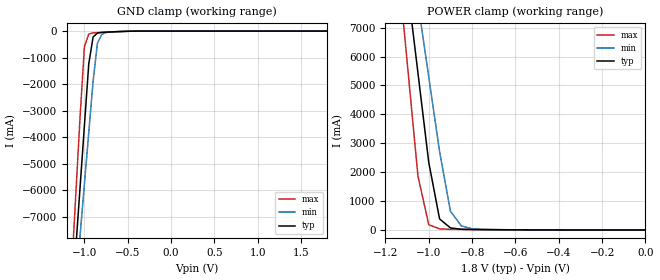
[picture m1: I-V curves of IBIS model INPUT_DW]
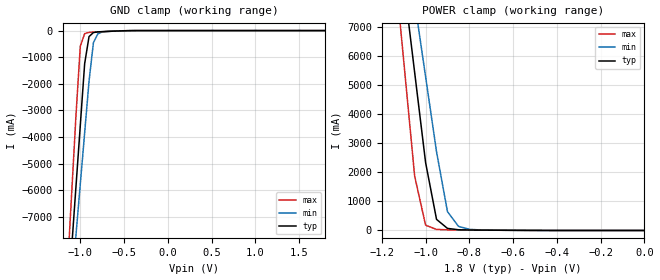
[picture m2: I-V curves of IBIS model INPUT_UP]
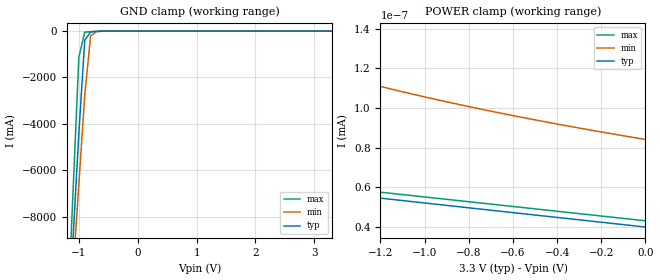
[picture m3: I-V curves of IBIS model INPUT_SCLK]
|   PERICOM SEMICONDUCTOR CORP
|   IBIS Model of PI6CG18801
|   Product Family: 6CG
|   TQFN 48-Pins (ZL) Package
[IBIS Ver] 3.2
[Comment char] |_char
[File Name] pi6cg18801_zl_reva.ibs
[File Rev] 1.0
[Source] File originated at Pericom Semiconductor Corp.
[Date] 12/20/16
[Disclaimer] (C) Copyright PERICOM Semiconductor Corporation
   All rights reserved
  Pericom Semiconductor Corporation hereby grants the user of
  this IBIS model a non-exclusive,nontransferable license to
  use this IBIS model under the following terms.
  This IBIS model is provided on an "AS IS" basis and Pericom
  makes absolutely no warranty with respect to the information
  contained herein. PERICOM DISCLAIMS AND CUSTOMER WAIVES ALL
  WARRANTIES,EXPRESSED OR IMPLIED,INCLUDING WARRANTIES OF
  MERCHANTABILITY OR FITNESS FOR A PARTICULAR PURPOSE. The
  entire risk as to quality and performance is with the customer.
  Accordingly,in no event shall the company be liable for any
  damages,whether in contract or tort,including any lost
  profits or other incidental,consequential,exemplary,or
  punitive damages arising out of the use or application of the
  IBIS model provided in this package. Further,Pericom reserves
  the right to make changes without notice to any product herein
  to improve reliability,function,or design. Pericom does not
  convey any license under patent rights or any other intellectual
  property rights,including those of third parties.
  The user is granted this license only to use the IBIS model
  and is not granted rights to sell,load,rent,lease or license
  the IBIS model in whole or in part,or in modified form to anyone
  other than user. User may modify the IBIS model to suit its specific
  application but rights to derivative works and such modifications
  shall belong to Pericom.
  Pericom is not obligated to provide maintenance or support
  for the licensed IBIS model.
  Contact Pericom at ATTN: APPLICATION ENGINEERING / IBIS MODELS
  1545 Barber Lane Milpitas,CA 95035 USA.
[Component] PI6CG18801
[Manufacturer] Pericom Semiconductor Corp.
[Package]
| Variable   typ   min   max
R_pkg   0.03902ohm   0.02922ohm   0.04882ohm
L_pkg   0.79998nH   0.76828nH   0.83168nH
C_pkg   0.19606pF   0.17176pF   0.22036pF
[Pin]  signal_name   model_name   R_pin   L_pin   C_pin
1   SS_EN_TRI   INPUT_DW   0.04882   0.83168nH   0.22036pF
2   GND_XTAL   GND   0.04490   0.81900nH   0.21064pF
3   XTAL_IN/CLK   NC   0.04098   0.80632nH   0.20092pF
4   XTAL_OUT   NC   0.03706   0.79364nH   0.19120pF
5   VDD_OSC   POWER   0.03314   0.78096nH   0.18148pF
6   VDD_REFOUT   POWER   0.02922   0.76828nH   0.17176pF
7   SDAR/REFOUT   REF_OUT   0.02922   0.76828nH   0.17176pF
8   GND_REFOUT   GND   0.03314   0.78096nH   0.18148pF
9   GND_DIG   GND   0.03706   0.79364nH   0.19120pF
10   SCLK   INPUT_SCLK   0.04098   0.80632nH   0.20092pF
11   SDATA   IO   0.04490   0.81900nH   0.21064pF
12   VDD_DIG   POWER   0.04882   0.83168nH   0.22036pF
13   VDDO   POWER   0.04882   0.83168nH   0.22036pF
14   OE0#   INPUT_DW   0.04490   0.81900nH   0.21064pF
15   Q0+   HCSL_OUT   0.04098   0.80632nH   0.20092pF
16   Q0-   HCSL_OUT   0.03706   0.79364nH   0.19120pF
17   OE1#   INPUT_DW   0.03314   0.78096nH   0.18148pF
18   Q1+   HCSL_OUT   0.02922   0.76828nH   0.17176pF
19   Q1-   HCSL_OUT   0.02922   0.76828nH   0.17176pF
20   VDD   POWER   0.03314   0.78096nH   0.18148pF
21   VDDO   POWER   0.03706   0.79364nH   0.19120pF
22   GND   GND   0.04098   0.80632nH   0.20092pF
23   Q2+   HCSL_OUT   0.04490   0.81900nH   0.21064pF
24   Q2-   HCSL_OUT   0.04882   0.83168nH   0.22036pF
25   OE2#   INPUT_DW   0.04882   0.83168nH   0.22036pF
26   Q3+   HCSL_OUT   0.04490   0.81900nH   0.21064pF
27   Q3-   HCSL_OUT   0.04098   0.80632nH   0.20092pF
28   OE3#   INPUT_DW   0.03706   0.79364nH   0.19120pF
29   GNDA   GND   0.03314   0.78096nH   0.18148pF
30   VDDA   POWER   0.02922   0.76828nH   0.17176pF
31   VDDO   POWER   0.02922   0.76828nH   0.17176pF
32   Q4+   HCSL_OUT   0.03314   0.78096nH   0.18148pF
33   Q4-   HCSL_OUT   0.03706   0.79364nH   0.19120pF
34   OE4#   INPUT_DW   0.04098   0.80632nH   0.20092pF
35   Q5+   HCSL_OUT   0.04490   0.81900nH   0.21064pF
36   Q5-   HCSL_OUT   0.04882   0.83168nH   0.22036pF
37   OE5#   INPUT_DW   0.04882   0.83168nH   0.22036pF
38   VDD   POWER   0.04490   0.81900nH   0.21064pF
39   VDDO   POWER   0.04098   0.80632nH   0.20092pF
40   GND   GND   0.03706   0.79364nH   0.19120pF
41   Q6+   HCSL_OUT   0.03314   0.78096nH   0.18148pF
42   Q6-   HCSL_OUT   0.02922   0.76828nH   0.17176pF
43   OE6#   INPUT_DW   0.02922   0.76828nH   0.17176pF
44   Q7+   HCSL_OUT   0.03314   0.78096nH   0.18148pF
45   Q7-   HCSL_OUT   0.03706   0.79364nH   0.19120pF
46   OE7#   INPUT_DW   0.04098   0.80632nH   0.20092pF
47   VDDO   POWER   0.04490   0.81900nH   0.21064pF
48   PD#   INPUT_UP   0.04882   0.83168nH   0.22036pF
[Diff Pin] inv_pin vdiff  tdelay_typ tdelay_min tdelay_max
6   7   NA   NA   NA   NA
3   4   NA   NA   NA   NA
15   16   NA   NA   NA   NA
18   19   NA   NA   NA   NA
23   24   NA   NA   NA   NA
26   27   NA   NA   NA   NA
32   33   NA   NA   NA   NA
35   36   NA   NA   NA   NA
41   42   NA   NA   NA   NA
44   45   NA   NA   NA   NA
[Model selector] REF_OUT
CMOS_SLOWEST  CMOS Output,REFSLEWRATE=0.9v/ns,slowest,slew_rate=00
CMOS_SLOW   CMOS Output,REFSLEWRATE=1.3v/ns,slow,slew_rate=01
CMOS_FAST   CMOS Output,REFSLEWRATE=1.6v/ns,fast,slew_rate=10
CMOS_FASTEST  CMOS Output,REFSLEWRATE=1.8v/ns,fastest,slew_rate=11
[Model selector] HCSL_OUT
HCSL_0P6_SLOW  Diff Output,Amplitude=0.6V,SMBUS=2v/ns,slow,slew_rate=0
HCSL_0P6_FAST  Diff Output,Amplitude=0.6V,SMBUS=3v/ns,fast,slew_rate=1
HCSL_0P7_SLOW  Diff Output,Amplitude=0.7V,SMBUS=2v/ns,slow,slew_rate=0
HCSL_0P7_FAST  Diff Output,Amplitude=0.7V,SMBUS=3v/ns,fast,slew_rate=1
HCSL_0P8_SLOW  Diff Output,Amplitude=0.8V,SMBUS=2v/ns,slow,slew_rate=0
HCSL_0P8_FAST  Diff Output,Amplitude=0.8V,SMBUS=3v/ns,fast,slew_rate=1
HCSL_0P9_SLOW  Diff Output,Amplitude=0.9V,SMBUS=2v/ns,slow,slew_rate=0
HCSL_0P9_FAST  Diff Output,Amplitude=0.9V,SMBUS=3v/ns,fast,slew_rate=1
| Models and submodels in the file (16): INPUT_DW (Input), INPUT_UP (Input), INPUT_SCLK (Input), CMOS_SLOWEST (Output), CMOS_SLOW (Output), CMOS_FAST (Output), CMOS_FASTEST (Output), IO (I/O_open_drain), HCSL_0P6_FAST (Output), HCSL_0P6_SLOW (Output), HCSL_0P7_FAST (Output), HCSL_0P7_SLOW (Output), HCSL_0P8_FAST (Output), HCSL_0P8_SLOW (Output), HCSL_0P9_FAST (Output), HCSL_0P9_SLOW (Output)
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|   Model INPUT_DW
[Model] INPUT_DW
Model_type Input
Vinl = 540.00mV
Vinh = 1.2600V
| variable   typ   min   max
C_comp   1.000pF   0.997pF   2.003pF
[Voltage Range]   1.8000V   1.7000V   1.9000V
[POWER Clamp Reference]   1.8000V   1.7000V   1.9000V
[GND Clamp Reference]   0.0000V   0.0000V   0.0000V
[Temperature Range]   25   85   -40
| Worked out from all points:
|   GND clamp passes 1 mA (typ) near -0.38 V on its own axis
|   POWER clamp passes 1 mA (typ) near -0.45 V on its own axis
[GND Clamp]
| Voltage   I(typ)   I(min)   I(max)
-1.8V     -40.8A     -36.77A    -47.86A
-1.15V    -10.55A    -11.59A    -9.184A
-1.1V     -8.222A    -9.649A    -6.209A
-1.05V    -5.896A    -7.712A    -3.234A
-1V       -3.569A    -5.775A    -591.1mA
-950mV    -1.243A    -3.838A    -113.6mA
-900mV    -226.2mA   -1.902A    -67.1mA
-850mV    -74.82mA   -458.6mA   -57.31mA
-800mV    -48.93mA   -124.4mA   -50.76mA
-750mV    -40.11mA   -53.69mA   -43.2mA
-350mV    -373.5uA   -930.2uA   -77.22uA
1.8V      14.98uA    16.02uA    13.77uA
[POWER Clamp]
| Voltage   I(typ)   I(min)   I(max)
-1.8V     52A        46.64A     61.4A
-1.15V    11.65A     13.04A     9.805A
-1.1V     8.543A     10.46A     5.838A
-1.05V    5.441A     7.877A     1.87A
-1V       2.338A     5.294A     182.5mA
-950mV    382.2mA    2.711A     36.48mA
-900mV    71.62mA    649.3mA    21.69mA
-850mV    24.89mA    142.9mA    18.06mA
-800mV    16.15mA    40.17mA    15.32mA
-750mV    12.65mA    17.76mA    12.41mA
0V        14.98uA    14.91uA    14.54uA
|   Model INPUT_UP
[Model] INPUT_UP
Model_type Input
Vinl = 540.00mV
Vinh = 1.2600V
| variable   typ   min   max
C_comp   1.000pF   0.997pF   2.003pF
[Voltage Range]   1.8000V   1.7000V   1.9000V
[POWER Clamp Reference]   1.8000V   1.7000V   1.9000V
[GND Clamp Reference]   0.0000V   0.0000V   0.0000V
[Temperature Range]   25   85   -40
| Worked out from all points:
|   GND clamp passes 1 mA (typ) near -0.38 V on its own axis
|   POWER clamp passes 1 mA (typ) near -0.45 V on its own axis
[GND Clamp]
| Voltage   I(typ)   I(min)   I(max)
-1.8V     -40.8A     -36.77A    -47.86A
-1.15V    -10.55A    -11.59A    -9.184A
-1.1V     -8.222A    -9.649A    -6.209A
-1.05V    -5.896A    -7.712A    -3.234A
-1V       -3.569A    -5.775A    -591.1mA
-950mV    -1.243A    -3.838A    -113.7mA
-900mV    -226.2mA   -1.902A    -67.12mA
-850mV    -74.83mA   -458.6mA   -57.32mA
-800mV    -48.94mA   -124.4mA   -50.78mA
-750mV    -40.12mA   -53.71mA   -43.22mA
-350mV    -388.4uA   -945.1uA   -91.75uA
1.8V      1.6nA      1.152uA    -765nA
[POWER Clamp]
| Voltage   I(typ)   I(min)   I(max)
-1.8V     52A        46.64A     61.4A
-1.15V    11.65A     13.04A     9.805A
-1.1V     8.543A     10.46A     5.838A
-1.05V    5.441A     7.877A     1.87A
-1V       2.338A     5.294A     182.4mA
-950mV    382.2mA    2.711A     36.46mA
-900mV    71.6mA     649.3mA    21.68mA
-850mV    24.88mA    142.8mA    18.05mA
-800mV    16.13mA    40.15mA    15.31mA
-750mV    12.64mA    17.75mA    12.39mA
0V        1.6nA      43.78nA    28.91pA
|   Model INPUT_SCLK
[Model] INPUT_SCLK
Model_type Input
Vinl = 990.00mV
Vinh = 2.3100V
| variable   typ   min   max
C_comp   1.000pF   0.997pF   2.003pF
[Voltage Range]   3.3000V   3.0000V   3.6000V
[POWER Clamp Reference]   3.3000V   3.0000V   3.6000V
[GND Clamp Reference]   0.0000V   0.0000V   0.0000V
[Temperature Range]   25   85   -40
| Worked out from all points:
|   GND clamp passes 1 mA (typ) near -0.52 V on its own axis
|   POWER clamp passes 1 mA (typ) near -2.41 V on its own axis
[GND Clamp]
| Voltage   I(typ)   I(min)   I(max)
-3.3V     -110.4A    -94.87A    -136.7A
-1.2V     -13.62A    -14.27A    -12.9A
-1.1V     -9.015A    -10.43A    -7.011A
-1V       -4.408A    -6.598A    -1.127A
-900mV    -398.5mA   -2.763A    -46.09mA
-800mV    -34.09mA   -202.3mA   -27.12mA
-700mV    -13.65mA   -21.62mA   -12.43mA
3.3V      40.05pA    89.93pA    39.6pA
[POWER Clamp]
| Voltage   I(typ)   I(min)   I(max)
-3.3V     31.96A     18.04A     54A
-2.1V     1.794nA    176.3pA    444.5nA
-2V       101.8pA    138.5pA    3.374nA
-1.9V     63.98pA    133.4pA    90.6pA
-1.8V     61.96pA    129.7pA    64.98pA
-1.4V     57.04pA    116.6pA    60pA
-1V       52.17pA    105.6pA    55.2pA
-500mV    46.1pA     94.04pA    49.2pA
0V        40.05pA    84.16pA    43.2pA
